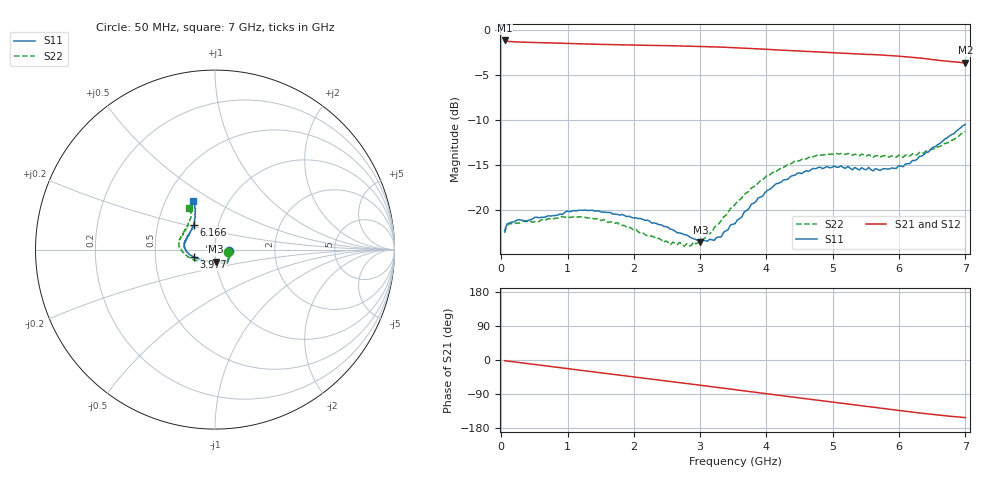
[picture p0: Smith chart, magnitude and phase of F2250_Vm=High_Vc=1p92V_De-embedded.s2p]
! Integrated Device Technology
! Corporate Headquarters
! 6024 Silver Creek Valley Road
! San Jose, CA 95138  USA
! Phone:  1-408-284-8200
! Toll Free:  1-800-223-1366
! Webpage:  http://www.idt.com/
! Timing and RF Division
! 515 Groton Road, Suite 102
! Westford, MA 01886-6024
! Device:  F2250
! Description: Voltage Variable RF Attenuator
! Frequency:  50.0 -  6000.00 MHz
! Package:  3x3 mm Thin QFN Plastic Package: 16 pin
! Ports:  2 RF, 3 DC
!  Pin  1  = GND
!  Pin  2  = NC
!  Pin  3  = RF1  = Port 1
!  Pin  4  = NC
!  Pin  5  = GND
!  Pin  6  = GND
!  Pin  7  = GND
!  Pin  8  = GND
!  Pin  9  = NC
!  Pin 10  = RF2  = Port 2
!  Pin 11  = NC
!  Pin 12  = GND
!  Pin 13  = GND
!  Pin 14  = VCNTRL
!  Pin 15  = VDD
!  Pin 16  = VMODE
! Vcntrl:  1.920 Volts
! Vmode:  +3.300 Volts
! Vdd:  +3.30  Volts
! Current:  1.323 mA
! Data:  The device was measured on a the F2250 evaluation board which has
!  individual transmission lines to the RF pins.  Data was collected
!  using a calibrated network analyzer.  The evaluation board was
!  de-embedded using a TRL calibration technique.
!  The reference plane is the edge of the package pin.
! Misc:  SN 10
!  Action Tracker AT0258
! Date Measured:  2014-11-26
! Date:  2015-10-15  MJV
! Note:
!  Integrated Device Technology supplies this data as a sample of measured
!  data at the package pin for this product.  Your particular data for this
!  product may vary.
!  Data was taken at 25 degrees C.
!  Integrated Device Technology reserves the right to change this data at anytime.
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# GHz S dB R 50
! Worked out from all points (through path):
!   201 points, 50 MHz to 7 GHz, reference 50 ohm
!   highest |S21| = -1.13 dB at 50 MHz (marker M1); lowest = -3.6 dB at 7 GHz (marker M2)
!   group delay of S21, straight-line fit = 61.1 ps
!   lowest |S11| = -23.5 dB at 3.004 GHz (marker M3), VSWR 1.14, Z = 50 - j6.68 ohm
!   |S11| at or under -10 dB: start of sweep to end of sweep
!   |S22| runs from -24.0 to -11.2 dB; largest |S21 - S12| = 0.0019
!   S11 on the Smith chart (normalised r, x): 50 MHz: 1.16, -0.02; 3.977 GHz: 0.79, -0.06; 6.166 GHz: 0.76, +0.22; 7 GHz: 0.68, +0.41
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0.05  -22.30 -7.4  -1.13 -1.8  -1.13 -1.8  -22.53 -8.3
0.08475  -21.54 -6.9  -1.22 -2.5  -1.21 -2.5  -21.70 -7.6
0.1195  -21.43 -7.6  -1.25 -3.3  -1.25 -3.3  -21.53 -7.4
0.6755  -20.73 -30.0  -1.39 -15.7  -1.39 -15.7  -21.07 -32.5
1.2315  -20.02 -48.0  -1.51 -27.9  -1.51 -27.9  -20.80 -55.2
1.75275  -20.47 -54.8  -1.61 -39.1  -1.61 -39.1  -21.39 -64.2
2.37825  -21.61 -56.6  -1.70 -52.7  -1.70 -52.7  -23.14 -70.8
2.552  -22.12 -60.4  -1.72 -56.5  -1.72 -56.6  -23.83 -77.3
2.7605  -22.72 -67.8  -1.75 -61.2  -1.75 -61.2  -24.00 -87.7
3.00375  -23.52 -85.9  -1.79 -66.7  -1.80 -66.7  -23.25 -107.1
3.1775  -23.29 -99.5  -1.83 -70.6  -1.83 -70.6  -22.43 -120.8
3.3165  -22.97 -116.8  -1.87 -73.8  -1.87 -73.8  -21.15 -131.0
3.4555  -21.67 -129.9  -1.91 -76.9  -1.91 -76.9  -19.82 -139.6
3.525  -21.51 -134.7  -1.94 -78.4  -1.94 -78.5  -19.39 -143.0
3.97675  -18.04 -161.3  -2.11 -88.6  -2.11 -88.7  -16.36 -163.8
4.4285  -16.11 -175.3  -2.28 -98.6  -2.29 -98.6  -14.53 -178.0
4.7065  -15.35 176.9  -2.38 -104.7  -2.39 -104.7  -14.07 175.8
5.054  -15.23 168.5  -2.51 -112.4  -2.51 -112.5  -13.69 168.3
5.85325  -15.42 141.8  -2.81 -129.9  -2.81 -130.0  -14.09 148.9
6.166  -14.79 130.1  -2.98 -136.8  -2.98 -136.8  -13.97 140.4
6.54825  -12.93 119.9  -3.28 -144.6  -3.29 -144.7  -13.15 128.2
7  -10.48 114.1  -3.61 -152.0  -3.62 -152.1  -11.25 121.6
